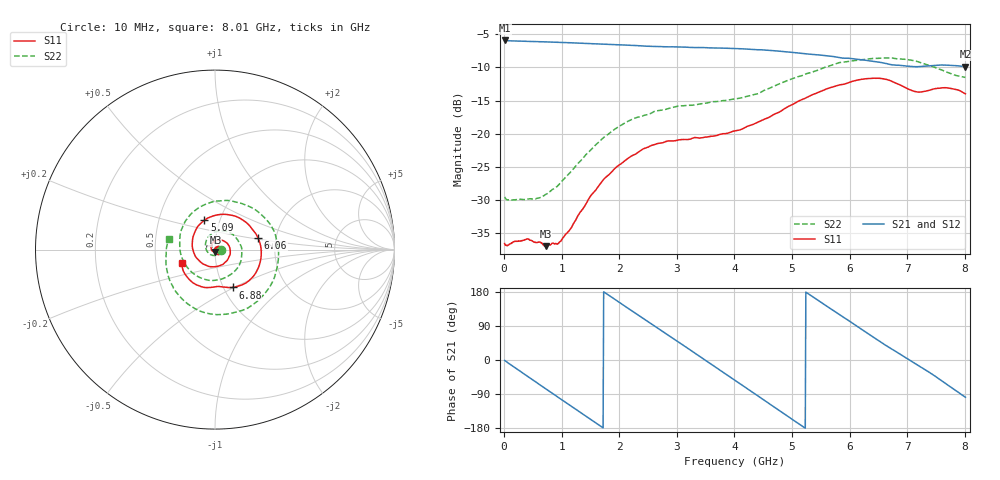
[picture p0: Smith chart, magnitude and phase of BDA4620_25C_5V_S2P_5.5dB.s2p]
!Agilent Technologies,E5071B,MY42404982,A.09.10
!Date: Wed May 06 08:59:16 2026
!Data & Calibration Information:
!Freq	S11:SOLT2(ON)	S21:SOLT2(ON)	S12:SOLT2(ON)	S22:SOLT2(ON)
# Hz S RI R 50
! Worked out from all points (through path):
!   801 points, 10 MHz to 8.01 GHz, reference 50 ohm
!   highest |S21| = -5.95 dB at 10 MHz (marker M1); lowest = -9.9 dB at 8.01 GHz (marker M2)
!   group delay of S21, straight-line fit = 284 ps
!   lowest |S11| = -36.9 dB at 720 MHz (marker M3), VSWR 1.03, Z = 50.2 - j1.41 ohm
!   |S11| at or under -10 dB: start of sweep to end of sweep
!   |S22| runs from -30.0 to -8.6 dB; largest |S21 - S12| = 0.0023
!   S11 on the Smith chart (normalised r, x): 10 MHz: 1.03, -0.00; 5.09 GHz: 0.84, +0.28; 6.06 GHz: 1.61, +0.23; 6.88 GHz: 1.10, -0.49; 8.01 GHz: 0.68, -0.10
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1e7  0.0149 -0.000862  0.5039 -0.0105  0.5048 -0.0109  0.0333 -0.00262
3.3e8  0.014 -0.00722  0.4081 -0.2843  0.4085 -0.2853  0.0217 -0.0234
7.2e8  0.0021 -0.0141  0.1221 -0.4763  0.1222 -0.4772  -0.0134 -0.0322
9.7e8  -0.0113 -0.0104  -0.0979 -0.4773  -0.0983 -0.4782  -0.0389 -0.0161
1.35e9  -0.0226 0.0139  -0.3733 -0.3024  -0.3736 -0.3029  -0.052 0.0374
1.65e9  -0.0118 0.0391  -0.4691 -0.0673  -0.4697 -0.0675  -0.0251 0.0831
1.94e9  0.015 0.0534  -0.4352 0.1725  -0.436 0.1728  0.0299 0.1053
2.32e9  0.0581 0.0425  -0.2256 0.4015  -0.2264 0.4021  0.1102 0.0747
2.68e9  0.0846 0.00139  0.0559 0.4504  0.0566 0.4507  0.1493 -0.00289
2.99e9  0.0772 -0.0445  0.2813 0.3524  0.2818 0.3521  0.1367 -0.0837
3.38e9  0.0347 -0.086  0.4367 0.0899  0.4374 0.0889  0.0506 -0.1589
3.69e9  -0.0163 -0.0955  0.4148 -0.1534  0.4141 -0.1547  -0.052 -0.1667
4.01e9  -0.0725 -0.0759  0.2608 -0.352  0.2604 -0.3525  -0.1499 -0.1051
4.51e9  -0.1266 0.0188  -0.1136 -0.4121  -0.1143 -0.4125  -0.1944 0.0834
5.09e9  -0.0598 0.1633  -0.3935 -0.1017  -0.394 -0.101  -0.00688 0.2675
5.35e9  0.0214 0.1953  -0.387 0.0826  -0.3872 0.0831  0.1231 0.2637
5.72e9  0.1533 0.1657  -0.2451 0.2919  -0.2448 0.2927  0.2875 0.1653
6.06e9  0.2401 0.0657  -0.0378 0.3651  -0.0372 0.3657  0.3542 -0.0164
6.68e9  0.1726 -0.1857  0.2782 0.1848  0.2794 0.1847  0.1904 -0.3203
6.88e9  0.0986 -0.2107  0.3158 0.0844  0.317 0.0838  0.0776 -0.3575
7.46e9  -0.0493 -0.2118  0.2488 -0.2111  0.2492 -0.2123  -0.223 -0.2276
8.01e9  -0.1855 -0.074  -0.0461 -0.3157  -0.0467 -0.3168  -0.2587 0.0587
